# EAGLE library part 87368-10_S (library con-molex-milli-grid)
RECEPTACAL
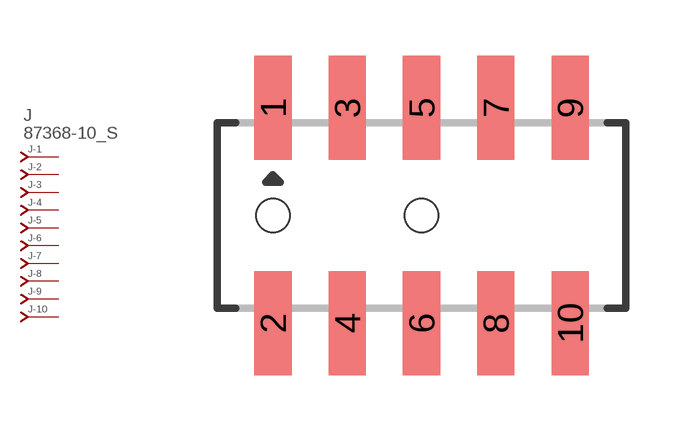
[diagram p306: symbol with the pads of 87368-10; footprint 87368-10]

Designator prefix J; gates -1=J-NV -2=J-N -3=J-N -4=J-N -5=J-N -6=J-N -7=J-N -8=J-N -9=J-N -10=J-N

## 87368-10_S  [87368-10]
1  -1:J  pas
2  -2:J  pas
3  -3:J  pas
4  -4:J  pas
5  -5:J  pas
6  -6:J  pas
7  -7:J  pas
8  -8:J  pas
9  -9:J  pas
10  -10:J  pas

## Footprint 87368-10 (pad centres in mm)
RECEPTACAL SMD Dual Row, Side Entry
smd 1 x 2.8: 1 -4,2.9; 2 -4,-2.9; 3 -2,2.9; 4 -2,-2.9; 5 0,2.9; 6 0,-2.9; 7 2,2.9; 8 2,-2.9; 9 4,2.9; 10 4,-2.9
hole 0.914 at -4,0
hole 0.914 at 0,0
